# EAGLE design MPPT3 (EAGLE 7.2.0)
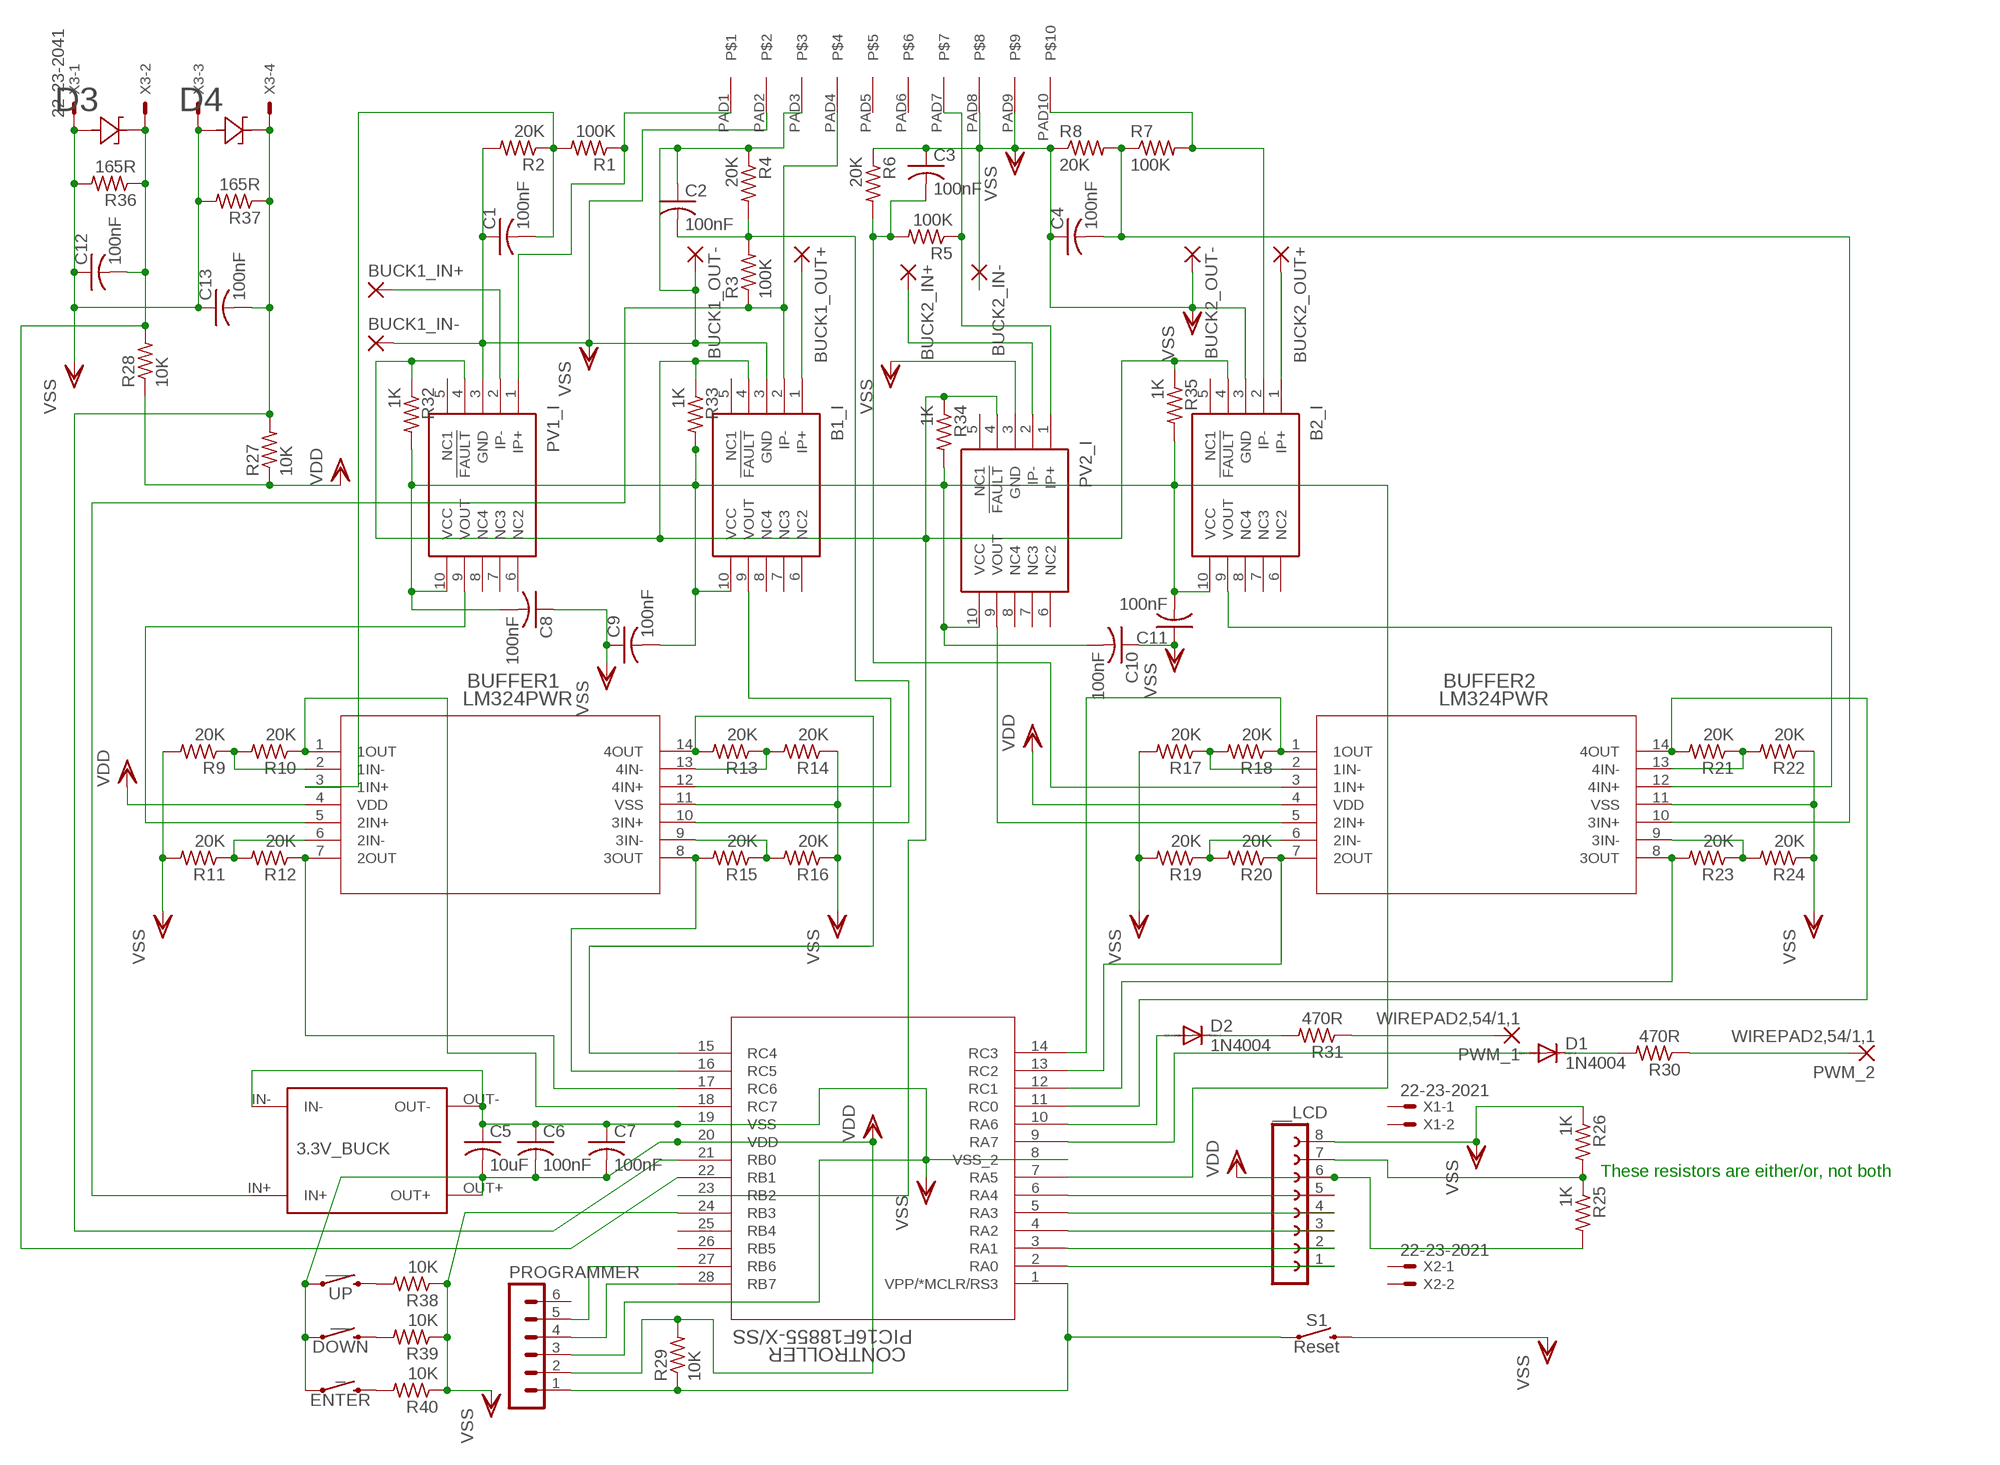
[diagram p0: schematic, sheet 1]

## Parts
3.3V_BUCK  TINY_BUCK  [TINY_BUCK]
_  ENTER  MOMENTARY-SWITCH-SPST-PTH-6.0MM  [TACTILE_SWITCH_PTH_6.0MM]
__  DOWN  MOMENTARY-SWITCH-SPST-PTH-6.0MM  [TACTILE_SWITCH_PTH_6.0MM]
___  UP  MOMENTARY-SWITCH-SPST-PTH-6.0MM  [TACTILE_SWITCH_PTH_6.0MM]
__LCD  FE08-1  [FE08]
B1_I  ACS711KEXLT-15AB-T  [EX-PACKAGE]
B2_I  ACS711KEXLT-15AB-T  [EX-PACKAGE]
BUCK1_IN+  3,81/1,4  [3,81/1,4]
BUCK1_IN-  3,81/1,4  [3,81/1,4]
BUCK1_OUT+  3,81/1,4  [3,81/1,4]
BUCK1_OUT-  3,81/1,4  [3,81/1,4]
BUCK2_IN+  3,81/1,4  [3,81/1,4]
BUCK2_IN-  3,81/1,4  [3,81/1,4]
BUCK2_OUT+  3,81/1,4  [3,81/1,4]
BUCK2_OUT-  3,81/1,4  [3,81/1,4]
BUFFER1  LM324PWR  [PW14]
BUFFER2  LM324PWR  [PW14]
C1  100nF  C-USC0603  [C0603]
C2  100nF  C-USC0603  [C0603]
C3  100nF  C-USC0603  [C0603]
C4  100nF  C-USC0603  [C0603]
C5  10uF  C-USC0603  [C0603]
C6  100nF  C-USC0603  [C0603]
C7  100nF  C-USC0603  [C0603]
C8  100nF  C-USC0603  [C0603]
C9  100nF  C-USC0603  [C0603]
C10  100nF  C-USC0603  [C0603]
C11  100nF  C-USC0603  [C0603]
C12  100nF  C-USC0603  [C0603]
C13  100nF  C-USC0603  [C0603]
CONTROLLER  PIC16F18855-X/SS  [SSOP28_MC]
D1  1N4004  [DO41-10]
D2  1N4004  [DO41-10]
D3  CZRU52C3V3  [CZRU]
D4  CZRU52C3V3  [CZRU]
PROGRAMMER  MA06-1  [MA06-1]
PV1_I  ACS711KEXLT-15AB-T  [EX-PACKAGE]
PV2_I  ACS711KEXLT-15AB-T  [EX-PACKAGE]
PWM_1  WIREPAD2,54/1,1  [2,54/1,1]
PWM_2  WIREPAD2,54/1,1  [2,54/1,1]
R1  100K  R-US_R0603  [R0603]
R2  20K  R-US_R0603  [R0603]
R3  100K  R-US_R0603  [R0603]
R4  20K  R-US_R0603  [R0603]
R5  100K  R-US_R1206  [R1206]
R6  20K  R-US_R0603  [R0603]
R7  100K  R-US_R0603  [R0603]
R8  20K  R-US_R0603  [R0603]
R9  20K  R-US_R0603  [R0603]
R10  20K  R-US_R0603  [R0603]
R11  20K  R-US_R0603  [R0603]
R12  20K  R-US_R0603  [R0603]
R13  20K  R-US_R0603  [R0603]
R14  20K  R-US_R0603  [R0603]
R15  20K  R-US_R0603  [R0603]
R16  20K  R-US_R0603  [R0603]
R17  20K  R-US_R0603  [R0603]
R18  20K  R-US_R0603  [R0603]
R19  20K  R-US_R0603  [R0603]
R20  20K  R-US_R0603  [R0603]
R21  20K  R-US_R0603  [R0603]
R22  20K  R-US_R0603  [R0603]
R23  20K  R-US_R0603  [R0603]
R24  20K  R-US_R0603  [R0603]
R25  1K  R-US_R0603  [R0603]
R26  1K  R-US_R0603  [R0603]
R27  10K  R-US_R1206  [R1206]
R28  10K  R-US_R0603  [R0603]
R29  10K  R-US_R0603  [R0603]
R30  470R  R-US_R0603  [R0603]
R31  470R  R-US_R1206  [R1206]
R32  1K  R-US_R1206  [R1206]
R33  1K  R-US_R1206  [R1206]
R34  1K  R-US_R0603  [R0603]
R35  1K  R-US_R0603  [R0603]
R36  165R  R-US_R0603  [R0603]
R37  165R  R-US_R0603  [R0603]
R38  10K  R-US_R0603  [R0603]
R39  10K  R-US_R0603  [R0603]
R40  10K  R-US_R0603  [R0603]
S1  Reset  MOMENTARY-SWITCH-SPST-PTH-6.0MM  [TACTILE_SWITCH_PTH_6.0MM]
U$1  CONN-KF2EDG-10(5.08)E-BAYPLUGGABLECONNECTORS  [CONN-KF2EDG-10(5.08)]
X1  22-23-2021  [22-23-2021]
X2  22-23-2021  [22-23-2021]
X3  22-23-2041  [22-23-2041]

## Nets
N$1: BUCK1_IN+.1(P) PV1_I.2(IP-)
N$2: BUFFER1.5(2IN+) PV1_I.9(VOUT)
N$3: BUFFER1.3(1IN+) C1.2 R1.2 R2.1
N$4: ___.3 R38.2
N$5: BUFFER1.10(3IN+) C2.2 R3.2 R4.2
N$6: 3.3V_BUCK.IN+ B1_I.2(IP-) R3.1 U$1.PAD4
N$7: B1_I.9(VOUT) BUFFER1.12(4IN+)
N$8: PV2_I.1(IP+) R5.1 U$1.PAD7
N$9: BUCK2_IN+.1(P) PV2_I.2(IP-)
N$10: __.3 R39.2
N$11: B2_I.2(IP-) R7.2 U$1.PAD10
N$12: BUFFER2.10(3IN+) C4.2 R7.1 R8.2
N$13: B2_I.1(IP+) BUCK2_OUT+.1(P)
N$14: BUFFER1.9(3IN-) R15.1 R16.2
N$15: BUFFER1.1(1OUT) CONTROLLER.18(RC7) R10.1
N$16: BUFFER1.6(2IN-) R11.1 R12.2
N$17: BUFFER1.7(2OUT) CONTROLLER.17(RC6) R12.1
N$18: BUFFER1.13(4IN-) R13.1 R14.2
N$19: BUFFER1.2(1IN-) R9.1 R10.2
N$20: BUFFER1.14(4OUT) CONTROLLER.15(RC4) R13.2
N$21: BUFFER1.8(3OUT) CONTROLLER.16(RC5) R15.2
N$22: B1_I.1(IP+) BUCK1_OUT+.1(P)
N$23: __LCD.1 CONTROLLER.2(RA0)
N$24: BUFFER2.1(1OUT) CONTROLLER.14(RC3) R18.1
N$25: BUFFER2.7(2OUT) CONTROLLER.13(RC2) R20.1
N$26: BUFFER2.6(2IN-) R19.1 R20.2
N$27: BUFFER2.14(4OUT) CONTROLLER.11(RC0) R21.2
N$28: BUFFER2.13(4IN-) R21.1 R22.2
N$29: BUFFER2.8(3OUT) CONTROLLER.12(RC1) R23.2
N$30: BUFFER2.9(3IN-) R23.1 R24.2
N$31: BUFFER2.2(1IN-) R17.1 R18.2
N$32: BUFFER2.5(2IN+) PV2_I.9(VOUT)
N$33: B2_I.9(VOUT) BUFFER2.12(4IN+)
N$34: __LCD.2 CONTROLLER.3(RA1)
N$35: __LCD.3 CONTROLLER.4(RA2)
N$36: __LCD.4 CONTROLLER.5(RA3)
N$37: __LCD.5 CONTROLLER.6(RA4)
N$38: __LCD.7 R25.1 R26.2
N$39: C12.2 CONTROLLER.22(RB1) D3.1 R28.2 R36.1 X3.2
N$40: CONTROLLER.1(VPP/*MCLR/RS3) PROGRAMMER.1 R29.1 S1.1
N$41: CONTROLLER.10(RA6) D2.A
N$42: C13.2 CONTROLLER.21(RB0) D4.1 R27.2 R37.1 X3.4
N$43: CONTROLLER.9(RA7) D1.A
N$44: CONTROLLER.28(RB7) PROGRAMMER.4
N$45: CONTROLLER.27(RB6) PROGRAMMER.5
N$46: PWM_2.1(P) R30.1
N$47: D1.C R30.2
N$48: PWM_1.1(P) R31.1
N$49: D2.C R31.2
N$50: PV1_I.1(IP+) R1.1 U$1.PAD1
N$51: _.3 R40.2
N$52: BUFFER2.3(1IN+) C3.2 R5.2 R6.2
N$53: B1_I.10(VCC) B2_I.10(VCC) C8.2 C9.2 C10.2 C11.2 CONTROLLER.7(RA5) PV1_I.10(VCC) PV2_I.10(VCC) R32.2 R33.2 R34.2 R35.2
N$56: B1_I.4(!FAULT) B2_I.4(!FAULT) CONTROLLER.23(RB2) PV1_I.4(!FAULT) PV2_I.4(!FAULT) R32.1 R33.1 R34.1 R35.1
VDD: 3.3V_BUCK.OUT+ _.1 __.1 ___.1 __LCD.6 BUFFER1.4(VDD) BUFFER2.4(VDD) C5.2 C6.2 C7.2 CONTROLLER.20(VDD) PROGRAMMER.2 R25.2 R27.1 R28.1 R29.2
VSS: 3.3V_BUCK.IN- 3.3V_BUCK.OUT- __LCD.8 B1_I.3(GND) B2_I.3(GND) BUCK1_IN-.1(P) BUCK1_OUT-.1(P) BUCK2_IN-.1(P) BUCK2_OUT-.1(P) BUFFER1.11(VSS) BUFFER2.11(VSS) C1.1 C2.1 C3.1 C4.1 C5.1 C6.1 C7.1 C8.1 C9.1 C10.1 C11.1 C12.1 C13.1 CONTROLLER.8(VSS_2) CONTROLLER.19(VSS) CONTROLLER.24(RB3) D3.2 D4.2 PROGRAMMER.3 PV1_I.3(GND) PV2_I.3(GND) R2.2 R4.1 R6.1 R8.1 R9.2 R11.2 R14.1 R16.1 R17.2 R19.2 R22.1 R24.1 R26.1 R36.2 R37.2 R38.1 R39.1 R40.1 S1.3 U$1.PAD2 U$1.PAD3 U$1.PAD8 U$1.PAD9 X3.1 X3.3
Unconnected: B1_I.5(NC1) B1_I.6(NC2) B1_I.7(NC3) B1_I.8(NC4) B2_I.5(NC1) B2_I.6(NC2) B2_I.7(NC3) B2_I.8(NC4) CONTROLLER.25(RB4) CONTROLLER.26(RB5) PROGRAMMER.6 PV1_I.5(NC1) PV1_I.6(NC2) PV1_I.7(NC3) PV1_I.8(NC4) PV2_I.5(NC1) PV2_I.6(NC2) PV2_I.7(NC3) PV2_I.8(NC4) U$1.PAD5 U$1.PAD6 X1.1 X1.2 X2.1 X2.2

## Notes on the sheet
- These resistors are either/or, not both

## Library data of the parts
3.3V_BUCK = Tiny_Buck:TINY_BUCK: E_Bay 3 Amp Buck Converter
_ __ ___ S1 = SparkFun-Switches:MOMENTARY-SWITCH-SPST: Momentary Switch (Pushbutton) - SPST; PROD_ID: SWCH-08441; SF_SKU: COM-00097
__LCD = con-lsta:FE08-1: FEMALE HEADER; OC_FARNELL: unknown; OC_NEWARK: unknown
B1_I B2_I PV1_I PV2_I = SamacSys_Parts:ACS711KEXLT-15AB-T: Hall Effect Linear Current Sensor with Overcurrent Fault Output for Source: Datasheet; ARROW_PART_NUMBER: ACS711KEXLT-15AB-T; DESCRIPTION: Hall Effect Linear Current Sensor with Overcurrent Fault Output for <100 V Isolation Applications; HEIGHT: mm; MANUFACTURER_NAME: Allegro Microsystems; MANUFACTURER_PART_NUMBER: ACS711KEXLT-15AB-T
BUCK1_IN+ BUCK1_IN- BUCK1_OUT+ BUCK1_OUT- BUCK2_IN+ BUCK2_IN- BUCK2_OUT+ BUCK2_OUT- = wirepad:3,81/1,4: THROUGH-HOLE PAD
BUFFER1 BUFFER2 = LM324PWR:LM324PWR; MANUFACTURER_PART_NUMBER: LM324PWR; VENDOR: Vendor
C1-C13 = resistor:C-US: CAPACITOR, American symbol
CONTROLLER = 16F18855_SSOP:PIC16F18855-X/SS; COPYRIGHT: Copyright (C) 2016 Accelerated Designs. All rights reserved; MANUFACTURER_PART_NUMBER: pic16f18855-x/ss; VENDOR: Microchip
D1 D2 = diode:1N4004: DIODE
D3 D4 = 0603ZenerDiode:CZRU52C3V3; VENDOR: Comchip
PROGRAMMER = con-lstb:MA06-1: PIN HEADER; OC_FARNELL: unknown; OC_NEWARK: unknown
PWM_1 PWM_2 = wirepad:WIREPAD: Wire PAD connect wire on PCB
R1-R26 R28-R40 = resistor:R-US_: RESISTOR, American symbol
R27 = rcl:R-US_: RESISTOR, American symbol
U$1 = Stuff_I_Use:CONN-KF2EDG-10(5.08)
X1 X2 = con-molex:22-23-2021: .100" (2.54mm) Center Header - 2 Pin; MF: MOLEX; MPN: 22-23-2021; OC_FARNELL: 1462926; OC_NEWARK: 25C3832
X3 = con-molex:22-23-2041: .100" (2.54mm) Center Header - 4 Pin; MF: MOLEX; MPN: 22-23-2041; OC_FARNELL: 1462920; OC_NEWARK: 38C0355

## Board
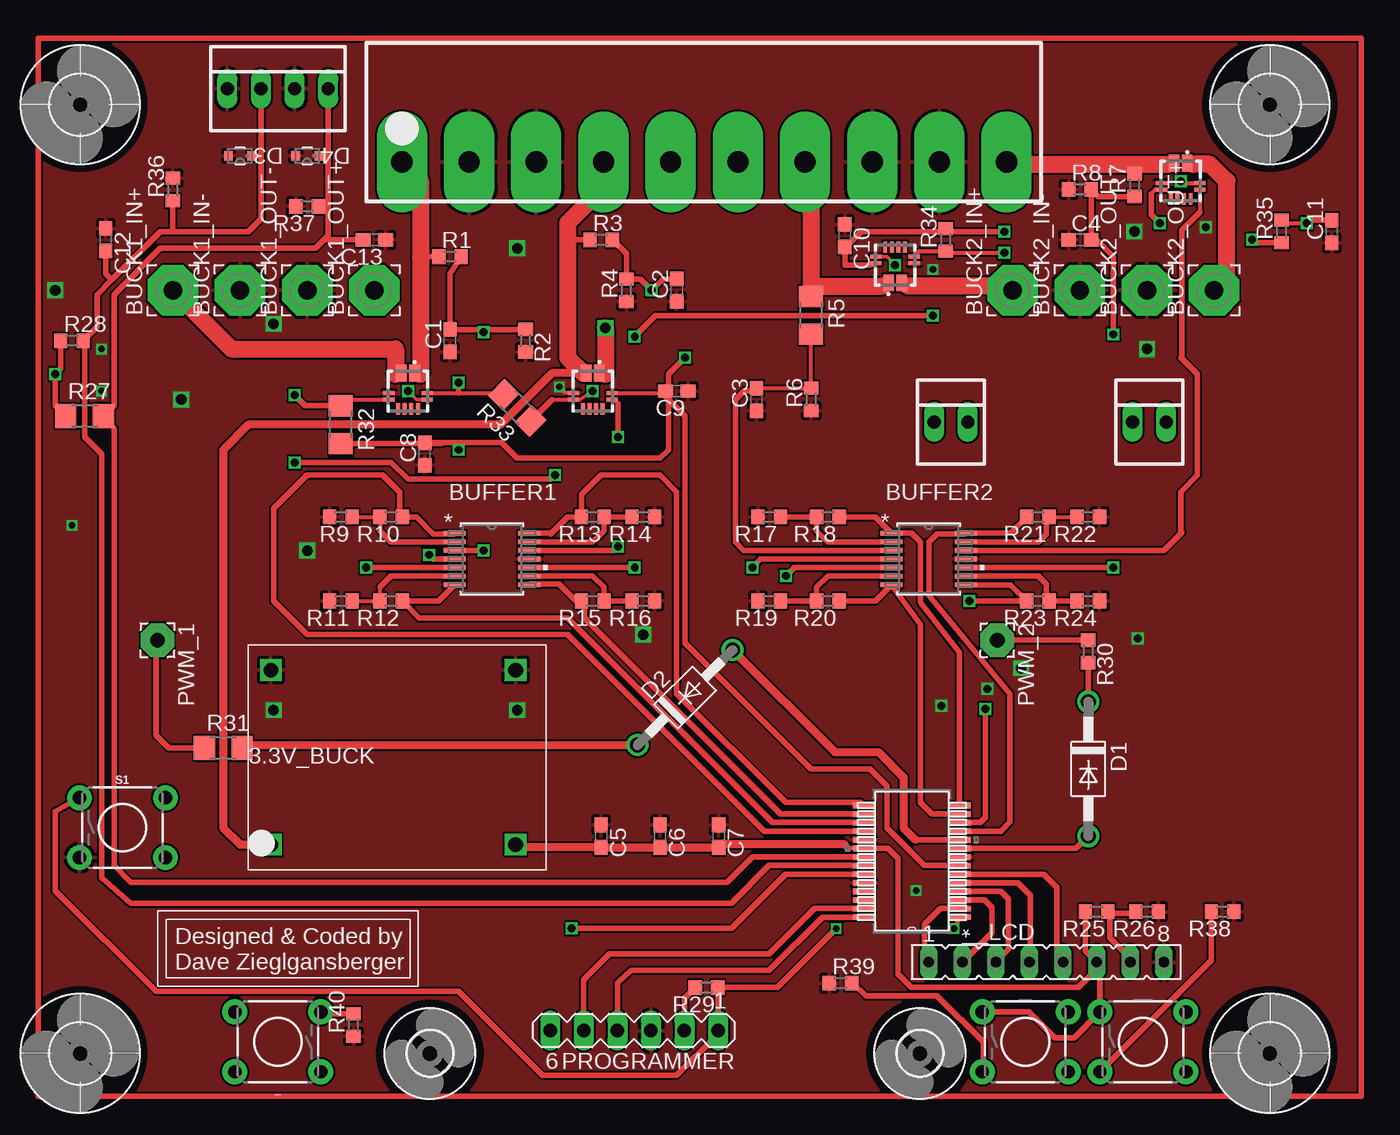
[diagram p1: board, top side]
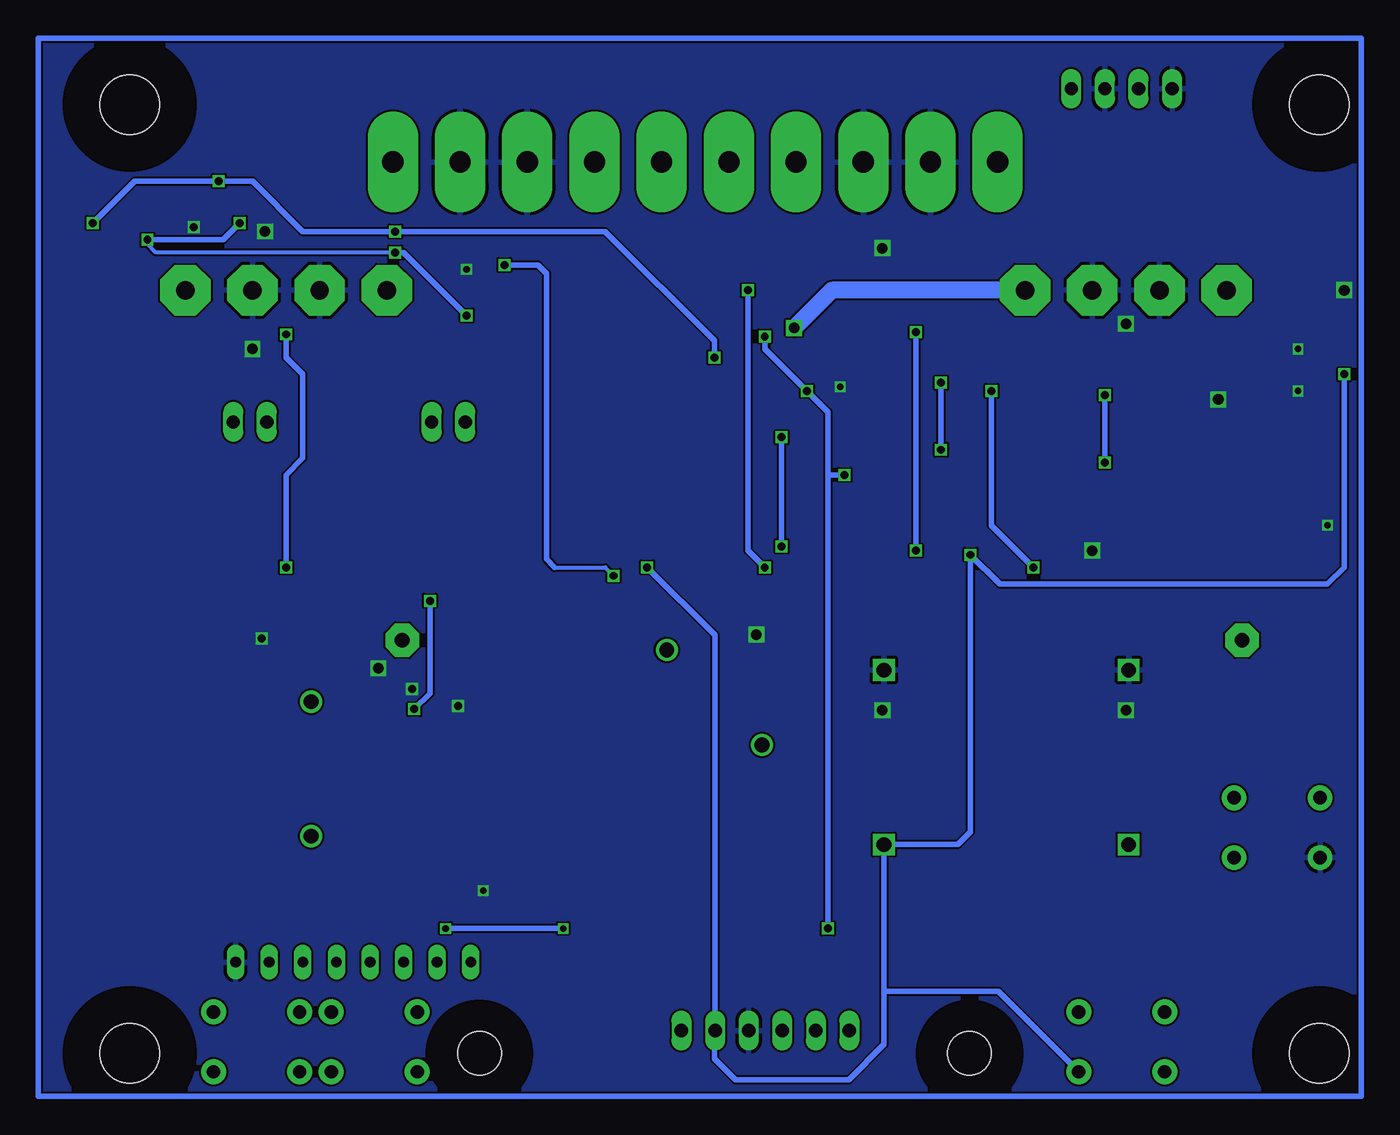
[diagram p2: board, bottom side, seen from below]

No outline drawn. Coordinates in mm, seen from the top.
Copper layers (1*16): Top 0.035mm / dielectric 1.5mm / Bottom 0.035mm
Design rules "SeeedStudio_2layer_DRU_no_angle_20140221 *": minimum track width 6mil, minimum drill 12mil, track to track 6mil, track to pad 6mil, pad to pad 6mil, via to via 6mil, smd to smd 0mil, copper to edge 10mil, drill to drill 10mil, minimum pad ring 10mil, minimum via ring 6mil, stop-mask expansion 2mil, vias tented up to drill 100mil, thermal gap 10mil

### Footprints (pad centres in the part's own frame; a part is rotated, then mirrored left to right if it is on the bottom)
TINY_BUCK = drill 1.1 square: IN+ 1.7,1.9; IN- 1.7,15.1; OUT+ 20.2,1.9; OUT- 20.2,15.1
TACTILE_SWITCH_PTH_6.0MM = drill 1.016 pad 1.88: 1 -3.251,2.261; 2 3.251,2.261; 3 -3.251,-2.261; 4 3.251,-2.261
FE08 = drill 0.813 long: 1 -8.89,0; 2 -6.35,0; 3 -3.81,0; 4 -1.27,0; 5 1.27,0; 6 3.81,0; 7 6.35,0; 8 8.89,0
EX-PACKAGE = smd 1.27 x 0.8: 1 -1.35,0.5; 2 -1.35,-0.5 | smd 0.3 x 0.85: 3 0.15,-1.45; 4 0.65,-1.45; 9 0.65,1.45; 10 0.15,1.45 | smd 0.85 x 0.3: 5 1.35,-0.75; 6 1.35,-0.25; 7 1.35,0.25; 8 1.35,0.75
3,81/1,4 = drill 1.397 pad 3.81 octagon: 1 0,0
PW14 = smd 1.676 x 0.356: 1 -2.819,1.95; 2 -2.819,1.3; 3 -2.819,0.65; 4 -2.819,0; 5 -2.819,-0.65; 6 -2.819,-1.3; 7 -2.819,-1.95; 8 2.819,-1.95; 9 2.819,-1.3; 10 2.819,-0.65; 11 2.819,0; 12 2.819,0.65; 13 2.819,1.3; 14 2.819,1.95
C0603 = smd 1.1 x 1: 1 -0.85,0; 2 0.85,0
SSOP28_MC = smd 1.676 x 0.432: 1 -3.619,4.225; 2 -3.619,3.575; 3 -3.619,2.925; 4 -3.619,2.275; 5 -3.619,1.625; 6 -3.619,0.975; 7 -3.619,0.325; 8 -3.619,-0.325; 9 -3.619,-0.975; 10 -3.619,-1.625; 11 -3.619,-2.275; 12 -3.619,-2.925; 13 -3.619,-3.575; 14 -3.619,-4.225; 15 3.619,-4.225; 16 3.619,-3.575; 17 3.619,-2.925; 18 3.619,-2.275; 19 3.619,-1.625; 20 3.619,-0.975; 21 3.619,-0.325; 22 3.619,0.325; 23 3.619,0.975; 24 3.619,1.625; 25 3.619,2.275; 26 3.619,2.925; 27 3.619,3.575; 28 3.619,4.225
DO41-10 = drill 1.118: A 5.08,0; C -5.08,0
CZRU = smd 0.66 x 0.711: 1 -0.876,0; 2 0.876,0
MA06-1 = drill 1.016 long: 1 -6.35,0; 2 -3.81,0; 3 -1.27,0; 4 1.27,0; 5 3.81,0; 6 6.35,0
2,54/1,1 = drill 1.118 pad 2.54 octagon: 1 0,0
R0603 = smd 1 x 1.1: 1 -0.85,0; 2 0.85,0
R1206 = smd 1.6 x 1.803: 1 -1.422,0; 2 1.422,0
CONN-KF2EDG-10(5.08) = drill 1.6 pad 3.81 long: PAD1 23.32,3; PAD2 18.24,3; PAD3 13.16,3; PAD4 8.08,3; PAD5 3,3; PAD6 -2.08,3; PAD7 -7.16,3; PAD8 -12.24,3; PAD9 -17.32,3; PAD10 -22.4,3
4,5 = hole 4.5: 0,0
3,3 = hole 3.3: 0,0
22-23-2021 = drill 1 long: 1 -1.27,0; 2 1.27,0
22-23-2041 = drill 1 long: 1 -3.81,0; 2 -1.27,0; 3 1.27,0; 4 3.81,0

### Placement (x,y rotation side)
3.3V_BUCK  15.88,17.14 0 top
_  18.1,4.13 180 top
__  74.61,4.13 0 top
___  83.5,4.13 0 top
__LCD  76.2,10.16 0 top
B1_I  41.91,53.34 270 top
B2_I  86.36,69.22 270 top
BUCK1_IN+  10.16,60.96 90 top
BUCK1_IN-  15.24,60.96 90 top
BUCK1_OUT+  25.4,60.96 90 top
BUCK1_OUT-  20.32,60.96 90 top
BUCK2_IN+  73.66,60.96 90 top
BUCK2_IN-  78.74,60.96 90 top
BUCK2_OUT+  88.9,60.96 90 top
BUCK2_OUT-  83.82,60.96 90 top
BUFFER1  34.29,40.64 0 top
BUFFER2  67.31,40.64 0 top
C1  31.11,57.15 90 top
C2  48.26,60.96 90 top
C3  54.29,52.7 90 top
C4  78.74,64.77 0 top
C5  42.55,19.68 270 top
C6  46.99,19.68 270 top
C7  51.44,19.68 270 top
C8  29.21,48.58 90 top
C9  48.26,53.34 180 top
C10  60.96,65.09 270 top
C11  97.79,65.41 90 top
C12  5.08,64.77 270 top
C13  25.4,64.77 180 top
CONTROLLER  66.04,17.78 180 top
D1  79.38,24.77 270 top
D2  48.9,30.16 45 top
D3  15.24,71.12 180 top
D4  20.32,71.12 180 top
PROGRAMMER  45.03,4.98 180 top
PV1_I  27.94,53.34 270 top
PV2_I  64.77,62.87 90 top
PWM_1  9,34.5 270 top
PWM_2  72.5,34.5 270 top
R1  31.11,63.5 0 top
R2  36.83,57.15 270 top
R3  42.55,64.77 0 top
R4  44.45,60.96 90 top
R5  58.42,59.05 270 top
R6  58.42,52.7 90 top
R7  82.87,68.9 90 top
R8  78.74,68.58 0 top
R9  22.86,43.81 180 top
R10  26.67,43.81 180 top
R11  22.86,37.47 180 top
R12  26.67,37.47 180 top
R13  41.91,43.81 180 top
R14  45.72,43.81 180 top
R15  41.91,37.47 180 top
R16  45.72,37.47 180 top
R17  55.24,43.81 180 top
R18  59.69,43.81 180 top
R19  55.24,37.47 180 top
R20  59.69,37.47 180 top
R21  75.56,43.81 180 top
R22  79.38,43.81 180 top
R23  75.56,37.47 180 top
R24  79.38,37.47 180 top
R25  80.01,13.97 180 top
R26  83.82,13.97 180 top
R27  3.49,51.44 0 top
R28  2.54,57.15 0 top
R29  50.52,8.24 180 top
R30  79.38,33.66 270 top
R31  13.97,26.35 0 top
R32  22.86,50.8 270 top
R33  36.2,52.07 135 top
R34  68.58,64.77 90 top
R35  93.98,65.41 90 top
R36  10.16,68.58 90 top
R37  20.32,67.31 180 top
R38  89.53,13.97 180 top
R39  60.64,8.57 0 top
R40  23.81,5.4 90 top
S1  6.35,20.32 0 top
U$1  50.8,73.66 180 top
U$2  [4,5]  3.15,75 0 top
U$3  [4,5]  93.1,3.25 0 top
U$4  [4,5]  3.15,3.25 0 top
U$5  [4,5]  93.1,75 0 top
U$7  [DAVE]  10.3,9.59 0 top
U$8  [3,3]  29.6,3.25 0 top
U$9  [3,3]  66.65,3.25 0 top
X1  69,51 0 top
X2  84,51 0 top
X3  18.1,76.2 0 top

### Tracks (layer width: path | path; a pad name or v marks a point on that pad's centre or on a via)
N$1
  Top 0.813: 26.99,54.61 27.07,54.69 PV1_I.2
  Top 1.27: BUCK1_IN+.1 14.61,56.52 26.99,56.52 26.99,54.61
N$2  (via drill 0.6)
  Top 0.254: v27.94,53.34 28.57,52.7 29.38,52.7 PV1_I.9
  Top 0.305: 31.46,40.01 BUFFER1.5
  Top 0.406: v24.77,40.01 31.46,40.01
  Bottom 0.406: v27.94,53.34 27.94,43.18 v24.77,40.01
N$3  (via drill 0.6)
  Top 0.305: 33.64,41.29 v33.66,41.27
  Top 0.406: 33.66,58 C1.2 31.11,62.23 R1.2 | 33.66,58 R2.1 | v33.66,57.78 33.66,58 | BUFFER1.3 31.49,41.27 v33.66,41.27
  Bottom 0.406: v33.66,41.27 v33.66,57.78
N$4
  Top 0.406: R38.2 88.69,10.3 ___.3
N$5  (via drill 0.6)
  Top 0.305: 37.12,40.01 BUFFER1.10
  Top 0.406: v45.09,40.01 37.12,40.01 | R3.2 44.45,63.72 R4.2 45.51,61.81 v46.35,60.96 47.2,61.81 C2.2
  Bottom 0.406: v46.35,60.96 46.35,41.27 v45.09,40.01
N$6
  Top 0.406: R3.1 40.01,64.77
  Top 0.61: 41.2,54.69 38.81,54.69 34.92,50.8 15.88,50.8 13.97,48.9 13.97,20.32 15.24,19.05 3.3V_BUCK.IN+
  Top 0.813: 41.2,54.69 B1_I.2
  Top 1.27: 41.2,54.69 40.01,55.88 40.01,64.77 40.01,66.04 42.72,68.75 U$1.PAD4
N$7  (via drill 0.6)
  Top 0.305: B1_I.9 43.51,52.69 43.81,52.39
  Top 0.406: BUFFER1.12 43.51,41.29 v43.81,41.59 | 43.81,52.39 v43.81,49.85
  Bottom 0.406: v43.81,41.59 v43.81,49.85
N$8
  Top 0.813: 63.82,61.28 64.06,61.52 PV2_I.1
  Top 1.27: 63.82,61.28 58.52,61.28 R5.1 58.42,70.2 U$1.PAD7
N$9
  Top 0.813: 65.72,61.28 65.48,61.52 PV2_I.2
  Top 1.27: BUCK2_IN+.1 73.34,61.28 65.72,61.28
N$10
  Top 0.406: __.3 71.44,1.94 71.44,4.13 67.94,7.62 62.55,7.62 61.59,8.57 R39.2
N$11
  Top 0.305: R7.2 82.55,70.06
  Top 0.406: R7.2 82.87,70.48
  Top 0.813: 85.41,70.48 85.49,70.56 B2_I.2
  Top 1.27: U$1.PAD10 73.38,70.48 82.87,70.48 85.41,70.48
N$12  (via drill 0.6)
  Top 0.305: 70.14,40.01 BUFFER2.10
  Top 0.406: v81.28,40.01 70.14,40.01 | v81.28,57.62 81.28,63.5 80.01,64.77 C4.2 R8.2 80.12,68.05 R7.1
  Bottom 0.406: v81.28,40.01 81.28,46.99 80.01,48.26 80.01,54.61 81.28,55.88 v81.28,57.62
N$13
  Top 0.813: 87.31,70.48 86.86,70.48 B2_I.1
  Top 1.27: BUCK2_OUT+.1 89.85,61.91 89.85,69.22 88.58,70.48 87.31,70.48
N$14
  Top 0.305: BUFFER1.9 37.14,39.37
  Top 0.406: 37.14,39.37 41.91,39.37 42.76,38.52 R15.1 R16.2
N$15
  Top 0.305: 31.43,42.55 BUFFER1.1 | 27.3,44.03 R10.1
  Top 0.406: R10.1 28.57,43.81 29.84,42.55 31.43,42.55 | CONTROLLER.18 54.88,20.05 40.01,34.92 20.32,34.92 17.78,37.47 17.78,44.45 20.32,46.99 26.04,46.99 27.3,45.72 27.3,44.03
N$16
  Top 0.305: R11.1 R12.2 25.82,38.52 | 31.44,39.37 BUFFER1.6
  Top 0.406: 25.82,38.52 26.67,39.37 31.44,39.37
N$17
  Top 0.305: 31.43,38.73 BUFFER1.7
  Top 0.406: BUFFER1.7 30.25,37.47 R12.1 28.79,36.2 40.01,36.2 55.49,20.7 CONTROLLER.17
N$18
  Top 0.305: 41.88,41.94 41.91,41.91
  Top 0.406: BUFFER1.13 41.88,41.94 | 41.91,41.91 42.76,42.76 R13.1 R14.2
N$19
  Top 0.305: R9.1 R10.2 25.82,42.76 | 31.44,41.91 BUFFER1.2
  Top 0.406: 25.82,42.76 26.67,41.91 31.44,41.91
N$20
  Top 0.305: 38.69,42.59 38.73,42.55 | 62.2,22.23 CONTROLLER.15
  Top 0.406: BUFFER1.14 38.69,42.59 | 38.73,42.55 40.01,43.81 R13.2 41.06,45.51 42.55,46.99 46.99,46.99 48.26,45.72 48.26,30.48 56.52,22.23 62.2,22.23
N$21
  Top 0.305: BUFFER1.8 37.15,38.73 | 40.64,37.47 R15.2 41.27,37.25
  Top 0.406: 37.15,38.73 39.37,38.73 40.64,37.47 | 41.27,37.25 41.27,36.2 56.12,21.36 CONTROLLER.16
N$22  (via drill 0.8)
  Top 0.813: 42.86,54.61 42.49,54.61 B1_I.1
  Top 1.27: v42.86,58.1 42.86,54.61
  Bottom 1.27: BUCK1_OUT+.1 40.01,60.96 v42.86,58.1
N$23
  Top 0.406: CONTROLLER.2 68.2,14.21 67,13 67,10.47 __LCD.1
N$24
  Top 0.305: 69.65,22.2 CONTROLLER.14
  Top 0.406: R18.1 63.27,43.81 BUFFER2.1 66,42.59 66.67,41.91 66.67,37.34 69.65,33.56 69.65,22.2
N$25
  Top 0.406: R20.1 63.27,37.47 BUFFER2.7 66.67,35.71 66.67,22.23 67.55,21.36 CONTROLLER.13
N$26
  Top 0.305: 64.46,39.37 BUFFER2.6
  Top 0.406: R19.1 R20.2 58.84,38.52 59.69,39.37 64.46,39.37
N$27
  Top 0.305: 70.08,42.55 BUFFER2.14
  Top 0.406: BUFFER2.14 73.49,42.59 R21.2 | CONTROLLER.11 72.76,20.05 73.46,20.75 73.46,30.42 67.31,37.87 67.31,41.91 67.94,42.55 70.08,42.55
N$28
  Top 0.305: 76.2,43.6 R21.1 R22.2
  Top 0.406: BUFFER2.13 75.59,41.94 76.2,42.55 76.2,43.6
N$29  (via drill 0.6)
  Top 0.406: BUFFER2.8 73.49,38.69 R23.2 v70.39,37.47 | CONTROLLER.12 71.2,20.7 71.59,21.09 v71.59,29.29
  Bottom 0.406: v71.59,29.29 70.39,30.48 v70.39,37.47
N$30
  Top 0.305: 76.2,37.68 R23.1
  Top 0.406: BUFFER2.9 75.59,39.34 76.2,38.73 76.2,37.68 | R23.1 R24.2
N$31
  Top 0.305: 64.46,41.91 BUFFER2.2
  Top 0.406: R17.1 R18.2 58.84,42.76 59.69,41.91 64.46,41.91
N$32  (via drill 0.6)
  Top 0.254: 63.34,63.5 64.14,63.5 v64.77,62.87
  Top 0.305: 64.48,40.01 BUFFER2.5 | PV2_I.9 63.34,63.5
  Top 0.406: v56.52,39.37 57.15,40.01 64.48,40.01
  Bottom 0.305: 60.96,40.01 57.15,40.01 v56.52,39.37
  Bottom 0.406: 60.96,40.01 61.59,40.64 61.59,62.23 62.23,62.87 v64.77,62.87
N$33
  Top 0.305: B2_I.9 87.81,66.86 | 70.14,41.27 BUFFER2.12
  Top 0.406: 87.81,66.86 86.46,65.5 86.46,55.98 86.36,55.88 87.63,54.61 87.63,46.99 86.36,45.72 86.36,42.74 86.46,42.65 85.09,41.27 70.14,41.27
N$34
  Top 0.406: CONTROLLER.3 71.5,14.86 72.07,14.29 72.07,12.38 __LCD.2
N$35
  Top 0.406: CONTROLLER.4 72.76,15.51 73.34,14.92 73.34,11.11 __LCD.3
N$36
  Top 0.406: CONTROLLER.5 74.07,16.16 75,15.22 75,10.23 __LCD.4
N$37
  Top 0.406: CONTROLLER.6 76,16.8 77,15.81 77,10.63 __LCD.5
N$38
  Top 0.406: __LCD.7 82.55,10.45 81,12 81,13.83 | 81,13.83 R25.1 | 81,13.83 82.83,13.83 R26.2
N$39
  Top 0.406: 5.56,61.75 9.21,65.41 10.16,65.41 | 5.56,61.75 4.45,60.64 4.45,58.2 R28.2 3.5,56.73 3.49,49.84 4.77,48.57 4.77,16.51 6.99,14.61 52.39,14.61 55.24,17.45 CONTROLLER.22 | 10.16,65.41 15.88,65.41 16.83,66.36 16.83,71.12 | 16.83,71.12 X3.2 | D3.1 16.83,71.12 | R36.1 10.16,65.41 | C12.2 5.08,62.23 5.56,61.75
N$40  (via drill 0.5)
  Top 0.305: CONTROLLER.1 v69.22,12.7
  Top 0.406: v60.33,12.7 55.88,8.26 R29.1 PROGRAMMER.1 51.38,4.71 48.26,1.59 38.1,1.59 31.75,7.94 8.89,7.94 1.27,15.56 1.27,21.55 S1.1
  Bottom 0.406: v69.22,12.7 v60.33,12.7
N$41
  Top 0.406: 66.32,19.41 CONTROLLER.10
  Top 0.61: D2.A 60.21,26.04 63.5,26.04 65.41,24.13 65.41,20.32 66.32,19.41
N$42
  Top 0.406: CONTROLLER.21 53.98,18.11 52.07,16.19 6.99,16.19 5.71,17.46 5.71,50.48 4.92,51.28 R27.2 5.71,52.24 5.71,60.64 9.21,64.14 20.95,64.14 21.59,64.77 | 21.59,64.77 21.91,65.09 21.91,67.31 | 21.91,67.31 21.91,71.12 | 21.91,71.12 X3.4 | D4.1 21.91,71.12 | R37.1 21.91,67.31 | C13.2 21.59,64.77
N$43
  Top 0.406: CONTROLLER.9 78.44,18.75 D1.A
N$44
  Top 0.406: CONTROLLER.28 59.27,13.55 55.24,9.53 44.8,9.53 43.77,8.59 PROGRAMMER.4
N$45
  Top 0.406: CONTROLLER.27 58.66,14.21 55.24,10.79 43.2,10.79 41.23,8.82 PROGRAMMER.5
N$46
  Top 0.406: R30.1 PWM_2.1
N$47
  Top 0.406: D1.C R30.2
N$48
  Top 0.406: R31.1 9.84,26.35 8.89,27.3 8.89,34.39 PWM_1.1
N$49
  Top 0.61: R31.2 15.61,26.57 D2.C
N$50
  Top 0.406: R1.1 28.89,63.5
  Top 0.813: 28.89,54.61 28.81,54.69 PV1_I.1
  Top 1.27: U$1.PAD1 28.89,69.25 28.89,63.5 28.89,54.61
N$51
  Top 0.406: _.3 21.49,6.25 R40.2
N$52
  Top 0.305: C3.2 R6.2 R5.2
  Top 0.406: BUFFER2.3 53.33,41.29 52.7,41.91 52.7,52.7 53.34,53.34 54.08,53.34 C3.2
N$53  (via drill 0.6)
  Top 0.305: 86.51,69.06 B2_I.10 | R35.2 94.19,66.04 v95.89,66.04 | 62.87,62.87 63.17,62.87 PV2_I.10 | PV1_I.10 31.75,53.19 35.19,53.19 R33.2 | B1_I.10 47.41,53.19 C9.2
  Top 0.406: C11.2 95.89,66.25 v95.89,66.04 | v86.36,69.22 86.51,69.06 | 62.87,62.87 60.96,62.87 C10.2 61.06,64.24 62.23,65.41 68.36,65.41 R34.2 68.8,65.41 v73.03,65.41 | R32.2 30.48,49.38 C8.2 31.8,49.43 | 31.8,49.43 35.03,49.43 36.2,48.26 46.99,48.26 47.62,48.9 47.62,53.12 | 47.62,53.12 C9.2 47.41,52.92 48.9,51.44 48.9,34.29 58.42,24.77 62.87,24.77 64.14,23.5 64.14,20.32 67,17.45 CONTROLLER.7 | 31.8,49.43 31.8,48.94 v31.75,48.9 | v31.75,53.98 31.75,53.19 | 47.62,53.12 47.62,54.61 v48.9,55.88
  Bottom 0.406: v95.89,66.04 92.71,69.22 v86.36,69.22 83.82,69.22 80.01,65.41 v73.03,65.41 57.15,65.41 48.9,57.15 v48.9,55.88 | v31.75,48.9 v31.75,53.98
N$54
  Bottom 0.406: 0,0 0,80 100,80 100,0 0,0
N$55
  Top 0.406: 0,0 0,80 100,80 100,0 0,0
N$56  (via drill 0.6)
  Top 0.254: B1_I.4 40.94,52.69 v41.91,53.34
  Top 0.305: B2_I.4 84.44,68.56 84.14,68.26 | 38.83,52.69 B1_I.4 | R32.1 23.33,52.69 PV1_I.4 | PV2_I.4 66.62,63.92 R34.1 68.68,63.82 v73.03,63.82
  Top 0.406: 84.14,68.26 84.14,66.67 v84.77,66.04 | R35.1 91.76,64.56 v91.76,64.77 | R33.1 38.83,52.69 | CONTROLLER.23 56.49,16.8 52.39,12.7 v40.32,12.7 | R32.1 20.17,52.22 v19.37,53.02 | v19.37,47.94 26.67,47.94 27.94,46.67 38.73,46.67 v39.05,46.99 | v45.09,57.47 46.67,59.05 v67.63,59.05
  Bottom 0.305: v73.03,63.82 91.12,63.82 91.76,64.45 v91.76,64.77
  Bottom 0.406: v84.77,66.04 86.04,64.77 v91.76,64.77 | v40.32,12.7 40.32,46.99 | 40.32,46.99 40.32,51.75 v41.91,53.34 45.09,56.52 v45.09,57.47 | v19.37,53.02 v19.37,47.94 | v39.05,46.99 40.32,46.99 | v67.63,59.05 72.39,63.82 v73.03,63.82
VDD  (via drill 0.6)
  Top 0.305: CONTROLLER.20 61.3,18.75 60.96,19.05
  Top 0.406: BUFFER1.4 29.84,40.64 v29.53,40.96 | R25.2 79.16,11.01 __LCD.6 | CONTROLLER.20 64.25,18.75 65,18 65,9.27 66,8.27 78.64,8.27 80.01,9.64 __LCD.6 | R28.1 1.69,55.03 v1.27,54.61 1.27,52.24 R27.1 | R29.2 48.84,7.42 PROGRAMMER.2 | BUFFER2.4 54.61,40.64 v53.98,40.01 | __LCD.6 80.25,9.92 ___.1 78.31,4.45 76.83,4.45 74.89,6.39 __.1
  Top 0.61: 60.96,19.05 51.85,19.05 C7.2 C6.2 C5.2 36.28,18.84 3.3V_BUCK.OUT+
  Bottom 0.406: 36.08,7.94 3.3V_BUCK.OUT+ 30.48,19.05 29.53,20 v29.53,40.96 27.3,38.73 2.54,38.73 1.27,40.01 v1.27,54.61 1.27,54.83 | 36.08,7.94 36.08,3.93 38.73,1.27 47.31,1.27 48.9,2.86 48.9,4.93 PROGRAMMER.2 48.84,34.88 v53.98,40.01 | _.1 27.42,7.94 36.08,7.94
VSS  (via drill 0.5, 0.6, 0.8)
  Top 0.305: B1_I.3 39.84,53.19 v39.37,53.66
  other vias: 20.32,41.27 82.87,65.41 83.82,56.52 1.27,60.96 17.78,58.42 45.72,34.92 17.78,29.21 36.2,29.21 4.76,56.52 4.76,53.34 88.27,65.72 83.14,34.63 68.26,29.53 2.54,43.18 36.2,64.14 10.79,52.7 74.3,32.38 71.75,30.8 66.36,15.56 67.63,62.55
  pour Bottom: 0,0 100,0 100,80 0,80
  pour Top: 0,80.01 100.33,80.01 100.33,0 0,0

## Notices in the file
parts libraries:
SparkFun-Switches: Licensing: Creative Commons ShareAlike 4.0 International - https://creativecommons.org/licenses/by-sa/4.0
